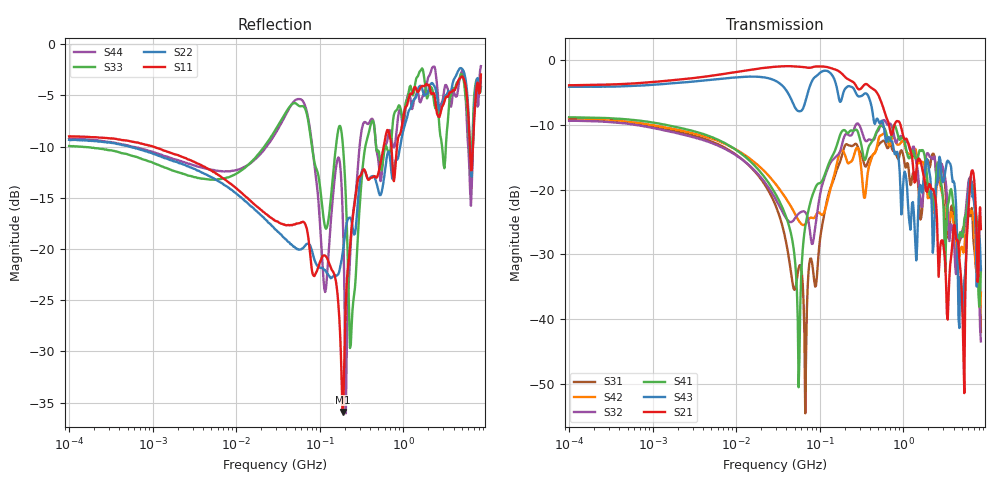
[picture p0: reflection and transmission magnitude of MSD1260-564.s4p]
# MHz S MA R 50
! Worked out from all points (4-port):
!   498 points, 100 kHz to 8.5 GHz, reference 50 ohm
!   strongest paths, dB at 100 kHz, 1.698 MHz, 29.49 MHz, 500.7 MHz, 8.5 GHz:
!     S21: -3.9, -3.1, -1.0, -5.3, -26.1
!     S43: -4.1, -3.6, -3.2, -9.3, -32.4
!     S41: -8.8, -10.2, -20.6, -10.6, -32.3
!     S32: -9.4, -11.1, -21.4, -10.9, -43.4
!     S42: -9.0, -10.6, -19.1, -12.4, -35.9
!     S31: -9.2, -10.8, -22.4, -13.2, -42.0
!   lowest |S11| = -35.9 dB at 187.5 MHz (marker M1), VSWR 1.03, Z = 51.3 + j0.943 ohm
!   |S11| at or under -10 dB: 1.023 MHz to 585.6 MHz (584.6 MHz wide, 199 % of centre); 721.5 MHz to 842.4 MHz (120.9 MHz wide, 15.5 % of centre); 6.268 GHz to 6.821 GHz (552.3 MHz wide, 8.44 % of centre)
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0.1  0.355 176.9  0.64 1.4  0.3485 -3.4  0.3624 -2.6
     0.64 1.4  0.3414 176.3  0.3407 -3.2  0.3552 -2.9
     0.3485 -3.4  0.3407 -3.2  0.3184 175.0  0.623 1.0
     0.3624 -2.6  0.3552 -2.9  0.623 1.0  0.3454 175.9
14.8634  0.172 110.2  0.8442 2.8  0.1498 -52.5  0.1648 -42.8
         0.8442 2.8  0.1624 131.1  0.1509 -37.7  0.1722 -35.9
         0.1498 -52.5  0.1509 -37.7  0.2643 81.4  0.7468 -6.1
         0.1648 -42.8  0.1722 -35.9  0.7468 -6.1  0.2623 92.1
55.89621  0.1336 45.3  0.8904 -12.0  0.02469 -20.6  0.002975 -53.5
          0.8904 -12.0  0.09943 89.5  0.06518 2.3  0.05767 -25.1
          0.02469 -20.6  0.06518 2.3  0.5012 -1.9  0.4039 -12.0
          0.002975 -53.5  0.05767 -25.1  0.4039 -12.0  0.5398 0.2
187.5231  0.01603 34.9  0.7792 -48.5  0.1915 44.5  0.2854 20.2
          0.7792 -48.5  0.09469 76.2  0.2314 32.2  0.1999 6.8
          0.1915 44.5  0.2314 32.2  0.3362 -61.9  0.532 -36.3
          0.2854 20.2  0.1999 6.8  0.532 -36.3  0.1568 -82.8
2260.241  0.575 175.8  0.1014 72.6  0.1896 126.7  0.08814 114.2
          0.1014 72.6  0.6423 -179.3  0.1724 119.2  0.08694 102.1
          0.1896 126.7  0.1724 119.2  0.587 160.4  0.03255 123.9
          0.08814 114.2  0.08694 102.1  0.03255 123.9  0.7752 172.5
5261.791  0.6819 -100.9  0.004988 40.9  0.05155 -138.4  0.04911 -105.4
          0.004988 40.9  0.7405 -108.7  0.04619 -106.0  0.03255 -135.4
          0.05155 -138.4  0.04619 -106.0  0.6719 -105.4  0.01045 -85.1
          0.04911 -105.4  0.03255 -135.4  0.01045 -85.1  0.7198 -112.6
8500  0.7112 -31.5  0.04958 -140.2  0.007966 -62.1  0.02437 -70.6
      0.04958 -140.2  0.686 -39.5  0.006723 -32.5  0.01606 -72.9
      0.007966 -62.1  0.006723 -32.5  0.6169 -37.5  0.02388 -147.0
      0.02437 -70.6  0.01606 -72.9  0.02388 -147.0  0.7813 -42.3
